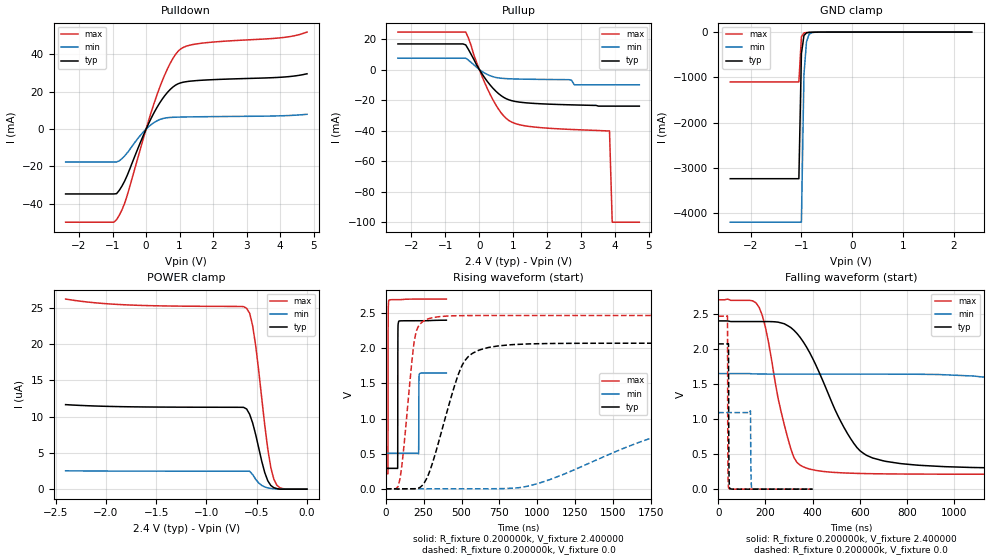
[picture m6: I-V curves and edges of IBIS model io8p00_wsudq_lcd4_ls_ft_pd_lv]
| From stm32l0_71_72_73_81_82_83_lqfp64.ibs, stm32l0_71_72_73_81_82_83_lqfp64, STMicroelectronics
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|   Model io8p00_wsudq_lcd4_ls_ft_pd_lv
[Model]  io8p00_wsudq_lcd4_ls_ft_pd_lv
Model_type I/O
Polarity   Non-Inverting
Enable   Active-Low
Vinl =   0.720000V
Vinh =   1.680000V
Vmeas =  1.200000V
Cref =   50.000000pF
Rref =   100.000000M
Vref =   0.0V
C_comp   3.178800pF   3.170000pF   3.206700pF
[Temperature Range]   25.000000   0.105000k   -40.000000
[Pullup Reference]   2.400000V   1.650000V   2.700000V
[Pulldown Reference]   0.0V   0.0V   0.0V
[POWER Clamp Reference]   2.400000V   1.650000V   2.700000V
[GND Clamp Reference]   0.0V   0.0V   0.0V
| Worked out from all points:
|   slope of the pulldown table from 0 to 0.36 V, typ, clamps not added: 28.5 ohm
|   slope of the pullup table from 0 to 0.36 V, typ, clamps not added: 32.2 ohm
|   GND clamp passes 1 mA (typ) near -0.64 V on its own axis
|   rising waveform, R_fixture 0.200000k, V_fixture 2.400000: 20-80 % time 734ps typ, 873ps min, 839ps max; typ from 0.291 V to 2.4 V
|   rising waveform, R_fixture 0.200000k, V_fixture 0.0: 20-80 % time 169ns typ, 820ns min, 66.4ns max; typ from 0 V to 2.07 V
|   falling waveform, R_fixture 0.200000k, V_fixture 2.400000: 20-80 % time 180ns typ, 729ns min, 89.7ns max; typ from 2.4 V to 0.291 V
|   falling waveform, R_fixture 0.200000k, V_fixture 0.0: 20-80 % time 1.26ns typ, 1.79ns min, 1.08ns max; typ from 2.07 V to 0 V
[Pulldown]
|Voltage   I(typ)   I(min)   I(max)
-2.4V     -34.71mA   -17.6mA    -49.82mA
-960mV    -34.71mA   -17.6mA    -49.82mA
-880mV    -34.55mA   -17.6mA    -48.46mA
-720mV    -30.52mA   -15.8mA    -43.27mA
-560mV    -24.65mA   -12.68mA   -35.33mA
0V        326fA      0A         10fA
400mV     13.84mA    5.066mA    22.03mA
720mV     21.25mA    6.254mA    35.26mA
1.04V     24.83mA    6.464mA    43.03mA
1.6V      26.11mA    6.627mA    45.88mA
4V        27.76mA    7.125mA    48.88mA
4.8V      29.63mA    7.94mA     51.96mA
[Pullup]
|Voltage   I(typ)   I(min)   I(max)
-2.4V     16.75mA    7.419mA    24.5mA
-400mV    16.1mA     7.419mA    24.5mA
0V        0A         0A         0A
320mV     -10.16mA   -4.078mA   -16.34mA
640mV     -17.08mA   -5.718mA   -28.28mA
960mV     -20.45mA   -6.128mA   -34.5mA
1.76V     -22.39mA   -6.47mA    -37.97mA
2.64V     -23.11mA   -6.64mA    -39.19mA
2.8V      -23.2mA    -10mA      -39.35mA
3.84V     -24mA      -10mA      -40.2mA
3.92V     -24mA      -10mA      -100mA
4.72V     -24mA      -10mA      -100mA
[GND_clamp]
|Voltage   I(typ)   I(min)   I(max)
-2.4V     -3.238A    -4.199A    -1.101A
-1.05V    -3.238A    -4.199A    -1.101A
-1V       -476.5mA   -4.199A    -104.7mA
-950mV    -76.69mA   -936.1mA   -18.75mA
-900mV    -16.87mA   -213.2mA   -9.366mA
-850mV    -6.718mA   -51.14mA   -6.786mA
-800mV    -4.121mA   -13.93mA   -5.004mA
-650mV    -1.082mA   -1.228mA   -1.183mA
2.35V     52.69uA    50.02uA    36.84uA
[POWER_clamp]
|Voltage   I(typ)   I(min)   I(max)
-2.4V     11.64uA    2.527uA    26.18uA
-1.86V    11.37uA    2.49uA     25.43uA
-600mV    11.04uA    2.475uA    24.9uA
-570mV    10.3uA     2.473uA    24.21uA
-540mV    9.097uA    2.001uA    22.48uA
-510mV    7.497uA    1.351uA    19.73uA
-450mV    3.846uA    513.2nA    12.52uA
-390mV    1.155uA    176.1nA    5.528uA
-360mV    508.6nA    103.4nA    2.997uA
-330mV    204.7nA    61.05nA    1.375uA
-270mV    0A         0A         195.3nA
0V        0A         0A         0A
[Ramp]
| variable   typ   min   max
dV/dt_r  0.65004/0.30188u   0.18965/0.80825u   1.03746/0.14375u
dV/dt_f  0.75702/0.32144u   0.19716/0.84573u   1.13800/0.15975u
R_load = 50.000000
[Rising Waveform]
R_fixture= 0.200000k
V_fixture= 2.400000
V_fixture_min= 1.650000
V_fixture_max= 2.700000
|time   V(typ)   V(min)   V(max)
0s        290.6mV    505.5mV    212.8mV
14.01ns   290.6mV    505.5mV    219.8mV
15.22ns   290.6mV    505.5mV    2.335V
19.62ns   290.6mV    505.5mV    2.68V
77.68ns   288.8mV    505.5mV    2.691V
79.68ns   2.203V     505.5mV    2.691V
84.08ns   2.376V     505.5mV    2.691V
216.2ns   2.391V     500.8mV    2.699V
222.2ns   2.391V     1.636V     2.699V
400ns     2.399V     1.648V     2.699V
[Rising Waveform]
R_fixture= 0.200000k
V_fixture= 0.0
V_fixture_min= 0.0
V_fixture_max= 0.0
|time   V(typ)   V(min)   V(max)
0s        2.004nV    12.6nV     1.54nV
93.43ns   -110uV     12.6nV     140.7mV
200.2ns   1.329mV    12.59nV    2.236V
280.3ns   196.6mV    -23.2uV    2.418V
360.4ns   755.4mV    -23.21uV   2.45V
533.9ns   1.854V     26.42uV    2.464V
840.8ns   2.051V     9.161mV    2.466V
1.909us   2.071V     821.4mV    2.466V
2.816us   2.071V     1.059V     2.466V
13.33us   2.071V     1.091V     2.466V
[Falling Waveform]
R_fixture= 0.200000k
V_fixture= 2.400000
V_fixture_min= 1.650000
V_fixture_max= 2.700000
|time   V(typ)   V(min)   V(max)
0s        2.399V     1.648V     2.699V
173.5ns   2.389V     1.642V     2.59V
307ns     2.305V     1.64V      580.9mV
520.5ns   955.6mV    1.64V      233.2mV
627.3ns   483.7mV    1.64V      221.9mV
840.8ns   343.1mV    1.638V     214.9mV
1.335us   297.2mV    1.497V     212.9mV
2.189us   290.8mV    721.2mV    212.8mV
2.936us   290.6mV    551.3mV    212.8mV
13.33us   290.6mV    505.5mV    212.8mV
[Falling Waveform]
R_fixture= 0.200000k
V_fixture= 0.0
V_fixture_min= 0.0
V_fixture_max= 0.0
|time   V(typ)   V(min)   V(max)
0s        2.071V     1.091V     2.466V
39.24ns   2.071V     1.091V     2.47V
41.24ns   2.071V     1.091V     306.5mV
43.64ns   2.07V      1.091V     27.36mV
44.84ns   728.2mV    1.091V     12.94mV
48.85ns   15.42mV    1.091V     2.667mV
136.5ns   28.81uV    1.117V     142.3uV
139.3ns   28.65uV    159.1mV    142.3uV
143.3ns   28.42uV    6.887mV    142.3uV
400ns     2.004nV    12.6nV     1.54nV
